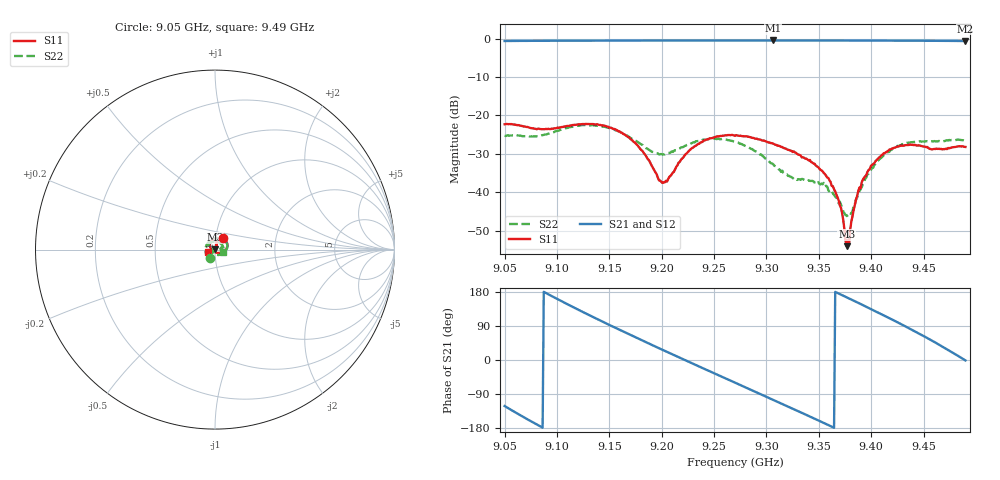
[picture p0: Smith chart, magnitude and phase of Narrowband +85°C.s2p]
!Agilent Technologies,N5230C,MY49001174,A.09.42.22
!Agilent N5230C: A.09.42.22
!Date: Friday, February 13, 2026 12:48:05
!Correction: S11(Full 2 Port(1,2))
!S21(Full 2 Port(1,2))
!S12(Full 2 Port(1,2))
!S22(Full 2 Port(1,2))
!S2P File: Measurements: S11, S21, S12, S22:
# Hz S  dB  R 50
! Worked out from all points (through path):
!   401 points, 9.05 GHz to 9.49 GHz, reference 50 ohm
!   highest |S21| = -0.49 dB at 9.3063 GHz (marker M1); lowest = -0.6 dB at 9.49 GHz (marker M2)
!   lowest |S11| = -54.0 dB at 9.3767 GHz (marker M3), VSWR 1.00, Z = 49.9 + j0.169 ohm
!   |S11| at or under -10 dB: start of sweep to end of sweep
!   |S22| runs from -46.5 to -22.5 dB; largest |S21 - S12| = 0.0018
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9.05e9  -22.32 56.9  -0.63 -121.4  -0.62 -121.4  -25.31 -120.2
9.0698e9  -22.93 49.6  -0.59 -153.4  -0.60 -153.4  -25.42 -179.2
9.0863e9  -23.60 49.9  -0.58 -178.5  -0.57 -178.5  -25.14 127.6
9.1039e9  -23.06 49.4  -0.56 155.8  -0.56 155.8  -23.73 80.5
9.1237e9  -22.30 39.1  -0.55 128.0  -0.54 128.0  -22.54 42.6
9.1589e9  -24.12 3.0  -0.53 80.8  -0.52 80.8  -24.23 -1.9
9.1798e9  -28.82 -28.5  -0.51 53.6  -0.51 53.6  -27.44 -12.1
9.1974e9  -36.91 -86.9  -0.51 31.1  -0.50 31.1  -30.15 0.9
9.204e9  -37.03 -136.3  -0.50 22.7  -0.50 22.7  -30.02 8.8
9.2326e9  -27.89 134.4  -0.50 -13.2  -0.50 -13.2  -26.74 11.6
9.27e9  -25.31 95.8  -0.50 -59.7  -0.50 -59.7  -26.88 -29.2
9.3063e9  -27.33 75.9  -0.49 -104.8  -0.50 -104.8  -32.65 -102.1
9.3437e9  -32.27 68.4  -0.50 -151.9  -0.50 -151.9  -37.04 125.6
9.3657e9  -39.81 66.8  -0.50 179.8  -0.50 179.8  -41.13 59.3
9.3767e9  -54.05 121.5  -0.51 165.4  -0.51 165.4  -45.96 -8.1
9.3866e9  -41.01 -152.4  -0.52 152.3  -0.51 152.3  -41.40 -88.3
9.3932e9  -36.25 -149.0  -0.52 143.5  -0.52 143.5  -37.33 -116.7
9.4174e9  -28.92 -164.5  -0.54 110.4  -0.54 110.4  -29.50 -175.9
9.435e9  -27.70 -173.4  -0.55 85.5  -0.55 85.4  -27.20 144.6
9.4515e9  -28.15 -175.4  -0.57 61.1  -0.57 61.1  -26.82 99.9
9.4724e9  -28.77 -159.6  -0.60 28.5  -0.60 28.4  -26.47 32.1
9.49e9  -28.22 -159.5  -0.64 -1.1  -0.63 -1.1  -26.70 -18.0
